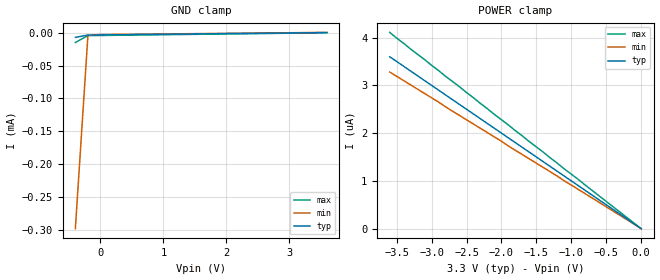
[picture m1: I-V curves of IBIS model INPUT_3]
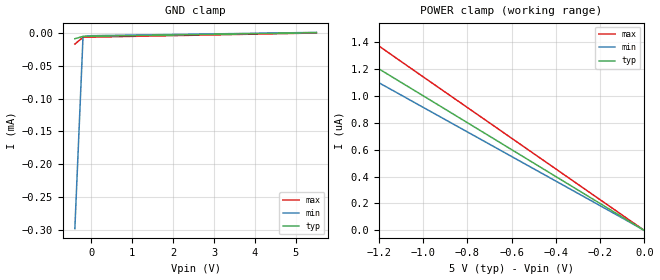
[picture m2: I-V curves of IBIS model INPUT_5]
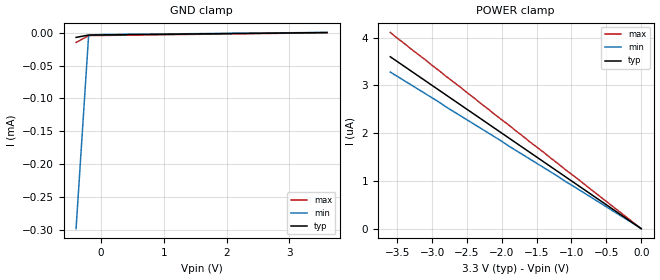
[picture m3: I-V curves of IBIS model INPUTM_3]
| Texas Instruments Incorporated
| Isolated Dual channel Buffer
| Marketing part#   Voltage Range   Package-type   #pins/pkg drawing
| ISO721D   3.0V - 5.5V   SOIC   8-pin D
| ISO721MD   3.0V - 5.5V   SOIC   8-pin D
| ISO722MD   3.0V - 5.5V   SOIC   8-pin D
[IBIS Ver]   4.1
[Comment char]   |_char
[File name]   iso721.ibs
[File Rev]   1.1
[Date]   05/02/2013
[Source]   Model built from spectre simulations at:
   Texas Instruments Incorporated.
   Analog-eLab, HPA
   12500 TI Blvd
   Dallas, TX -75243
   For Support e-mail: elab_ibis@list.ti.com
[Notes]   Revision History
   Rev 1.0: 22June07
   Rev 1.1: 05/02/2013
   -Update OUTPUT_5 and OUTPUT_3
   -Add 722, with enable to buffer model
   -Add CMOS input model
   - ccomp values are based on PVT settings:
   MIN: Low Voltage, High Temperature, Weak Process
   TYP: Nominal Voltage, Nominal Temperature, Nominal Process
   MAX: High Voltage, Low Temperature, Fast Process
   - C_comp although listed in numerical order of value are obtained from varying PVT conditions.
   For PVT conditions for each specific value, refer to the buffer description under respective [Model].
   IBIS model user is responsible for using appropriate C_comp to simulate for Signal Integrity.
[Disclaimer]  This model is designed as an aid for customers of Texas Instruments
 TI and its licensors and suppliers make no warranties, either expressed
 or implied, with respect to this  model, including the warranties of
 merchantability or fitness for a particular purpose.
 The model is provided solely on an "as is" basis. The entire risk as to
 its quality and performance is with the customer.
[Copyright] (C)Copyright 2013 Texas Instruments Incorporated.
   All rights reserved.
[Component]   ISO721D
[Manufacturer]  Texas Instruments Incorporated
[Package]
|   typ   min   max
R_pkg   0.055   0.034   0.067
L_pkg   1.795nH   1.699nH   1.914nH
C_pkg   0.299pF   0.278pF   0.311pF
[Pin]   signal_name   model_name   R_pin   L_pin   C_pin
1   VCC1   POWER   0.067   1.914n   0.278p
2   IN   INPUT   0.062   1.816n   0.301p
3   VCC1   POWER   0.053   1.699n   0.298p
4   GND1   GND   0.067   1.907n   0.278p
5   GND2   POWER   0.034   1.704n   0.311p
6   OUT   OUTPUT   0.061   1.808n   0.310p
7   GND2   GND   0.062   1.817n   0.302p
8   VCC2   POWER   0.034   1.716n   0.311p
[Component]   ISO722D
[Manufacturer]  Texas Instruments Incorporated
[Package]
|   typ   min   max
R_pkg   0.055   0.034   0.067
L_pkg   1.795nH   1.699nH   1.914nH
C_pkg   0.299pF   0.278pF   0.311pF
[Pin]   signal_name   model_name   R_pin   L_pin   C_pin
1   VCC1   POWER   0.067   1.914n   0.278p
2   IN   INPUT   0.062   1.816n   0.301p
3   VCC1   POWER   0.053   1.699n   0.298p
4   GND1   GND   0.067   1.907n   0.278p
5   GND2   POWER   0.034   1.704n   0.311p
6   OUT   OUTPUT   0.061   1.808n   0.310p
7   EN   ENABLE   0.062   1.817n   0.302p
8   VCC2   POWER   0.034   1.716n   0.311p
[Model Selector] INPUT
INPUT_3   3.3V TTL INPUT   ISO7221A, ISO7221B, ISO7221C Devices
INPUT_5   5.0V TTL INPUT   ISO7221A, ISO7221B, ISO7221C Devices
INPUTM_3   3.3V CMOS INPUT, ISO7221M device
INPUTM_5   5.0V CMOS INPUT  ISO7221M device
[Model Selector] ENABLE
ENABLE_3   3.3V OUTPUT
ENABLE_5   5.0V OUTPUT
[Model Selector] OUTPUT
OUTPUT_3   3.3V OUTPUT
OUTPUT_5   5.0V OUTPUT
| Models and submodels in the file (8): INPUT_3 (Input), INPUT_5 (Input), INPUTM_3 (Input), INPUTM_5 (Input), ENABLE_3 (Input), ENABLE_5 (Input), OUTPUT_3 (3-state), OUTPUT_5 (3-state)
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|   Input 3.3V Model
[Model]   INPUT_3
Model_type   Input
Vinh = 2.0
Vinl = 0.8
|   typ   min   max
C_comp   1.3pF   1.1pF   1.5pF
|   typ   min   max
[Temperature Range]   27   -40   125
[Voltage range]   3.3V   3.0V   3.6V
[GND_clamp]
|   Voltage   I(typ)   I(min)   I(max)
-400mV    -7.04uA    -298uA     -14.8uA
-200mV    -3.5uA     -3.91uA    -4.34uA
0V        -3.3uA     -2.74uA    -4.11uA
3.6V      300nA      549nA      14.4pA
[Power_clamp]
| Note that the[POWER_clamp]voltage table is referenced to Vcc
| and is calculated using Vtable=Vcc - Vmeasured.
|   Voltage   I(typ)   I(min)   I(max)
-3.6V     3.6uA      3.28uA     4.11uA
-2.9V     2.9uA      2.65uA     3.31uA
-2.8V     2.8uA      2.55uA     3.19uA
0V        0A         0A         0A
|   Input 5.0V Model
[Model]   INPUT_5
Model_type   Input
Vinh = 2.0
Vinl = 0.8
|   typ   min   max
C_comp   1.3pF   1.1pF   1.5pF
|   typ   min   max
[Temperature Range]   27   -40   125
[Voltage range]   5.0V   4.5V   5.5V
[GND_clamp]
|   Voltage   I(typ)   I(min)   I(max)
-400mV    -8.71uA    -298uA     -16.9uA
-200mV    -5.2uA     -5.27uA    -6.5uA
0V        -5uA       -4.1uA     -6.27uA
5.5V      500nA      913nA      27.5pA
[Power_clamp]
| Note that the[POWER_clamp]voltage table is referenced to Vcc
| and is calculated using Vtable=Vcc - Vmeasured.
|   Voltage   I(typ)   I(min)   I(max)
-5.5V     5.498uA    5.021uA    6.28uA
-1.7V     1.699uA    1.552uA    1.939uA
-1.6V     1.599uA    1.461uA    1.825uA
-1.5V     1.499uA    1.369uA    1.711uA
-1.4V     1.399uA    1.278uA    1.597uA
-1.3V     1.299uA    1.187uA    1.483uA
0V        0A         0A         0A
|   INPUTM_3 Model
[Model]   INPUTM_3
Model_type   Input
Vinl = 0.99
Vinh = 2.31
|   typ   min   max
C_comp   1.3pF   1.1pF   1.5pF
[Model Spec]
Vinl   0.99V   0.9V   1.08V
Vinh   2.31V   2.1V   2.52V
|   typ   min   max
[Temperature Range]   27   -40   125
[Voltage range]   3.3V   3.0V   3.6V
[GND_clamp]
|   Voltage   I(typ)   I(min)   I(max)
-400mV    -7.04uA    -298uA     -14.8uA
-200mV    -3.5uA     -3.91uA    -4.34uA
0V        -3.3uA     -2.74uA    -4.11uA
3.6V      300nA      549nA      14.4pA
[Power_clamp]
| Note that the[POWER_clamp]voltage table is referenced to Vcc
| and is calculated using Vtable=Vcc - Vmeasured.
|   Voltage   I(typ)   I(min)   I(max)
-3.6V     3.6uA      3.28uA     4.11uA
-2.9V     2.9uA      2.65uA     3.31uA
-2.8V     2.8uA      2.55uA     3.19uA
0V        0A         0A         0A
